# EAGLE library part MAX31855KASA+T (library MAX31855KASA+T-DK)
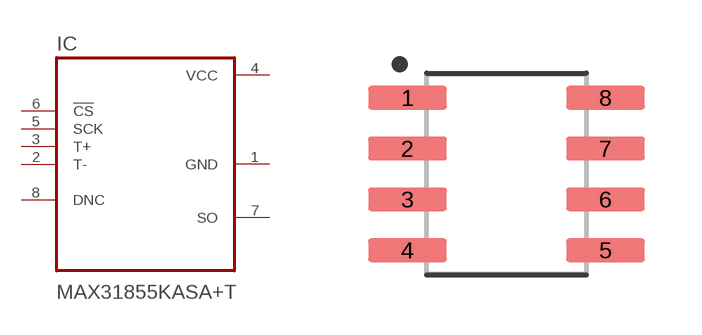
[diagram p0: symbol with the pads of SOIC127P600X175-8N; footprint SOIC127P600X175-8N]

Designator prefix IC

## MAX31855KASA+T  [SOIC127P600X175-8N]
1  GND  pas
2  T-  pas
3  T+  pas
4  VCC  pwr
5  SCK  in
6  !CS  in
7  SO  out
8  DNC  pas

## Footprint SOIC127P600X175-8N (pad centres in mm)
smd 1.97 x 0.59: 1 -2.475,1.905; 2 -2.475,0.635; 3 -2.475,-0.635; 4 -2.475,-1.905; 5 2.475,-1.905; 6 2.475,-0.635; 7 2.475,0.635; 8 2.475,1.905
